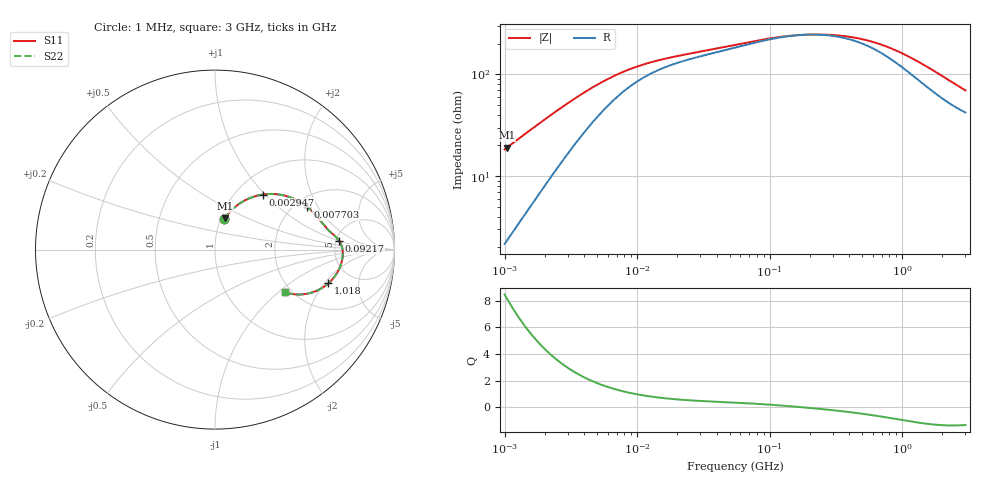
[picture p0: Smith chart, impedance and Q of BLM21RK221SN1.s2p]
! BLM21RK221SN1
# Hz S RI R 50
!Freq.(Hz) S11(Real) S11(Imag) S21(Real) S21(Imag) S12(Real) S12(Imag) S22(Real) S22(Imag)
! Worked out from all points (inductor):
!   401 points, 1 MHz to 3 GHz, reference 50 ohm
!   read as one part in series: L = 2.87 uH near 1.041 MHz
!   highest Q = 8.16 at 1.041 MHz (marker M1), where L = 2.89 uH
!   self-resonance near 183.6 MHz
!   S11 on the Smith chart (normalised r, x): 1 MHz: 1.04, +0.36; 2.947 MHz: 1.32, +0.97; 7.703 MHz: 2.32, +1.63; 92.17 MHz: 5.32, +1.01; 1.018 GHz: 3.31, -2.20; 3 GHz: 1.84, -1.11
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1000000  0.0512 0.169  0.9488 -0.169  0.9488 -0.169  0.0512 0.169
1040844  0.055 0.1747  0.945 -0.1747  0.945 -0.1747  0.055 0.1747
1751453  0.1324 0.2533  0.8676 -0.2533  0.8676 -0.2533  0.1324 0.2533
2947212  0.2674 0.307  0.7326 -0.307  0.7326 -0.307  0.2674 0.307
3823119  0.346 0.3083  0.654 -0.3083  0.654 -0.3083  0.346 0.3083
5481359  0.4448 0.2808  0.5552 -0.2808  0.5552 -0.2808  0.4448 0.2808
7703107  0.5144 0.2374  0.4856 -0.2374  0.4856 -0.2374  0.5144 0.2374
1.040059e7  0.5562 0.198  0.4438 -0.198  0.4438 -0.198  0.5562 0.198
1.461624e7  0.5881 0.16  0.4119 -0.16  0.4119 -0.16  0.5881 0.16
2.459509e7  0.6214 0.1192  0.3786 -0.1192  0.3786 -0.1192  0.6214 0.1192
5.477226e7  0.6653 0.0783  0.3347 -0.0783  0.3347 -0.0783  0.6653 0.0783
9.216659e7  0.6913 0.0493  0.3087 -0.0493  0.3087 -0.0493  0.6913 0.0493
2.094008e8  0.7115 -0.0106  0.2885 0.0106  0.2885 0.0106  0.7115 -0.0106
3.002264e8  0.7108 -0.0419  0.2892 0.0419  0.2892 0.0419  0.7108 -0.0419
4.219165e8  0.7038 -0.0759  0.2962 0.0759  0.2962 0.0759  0.7038 -0.0759
5.81181e8  0.6891 -0.1133  0.3109 0.1133  0.3109 0.1133  0.6891 -0.1133
8.005644e8  0.6625 -0.1554  0.3375 0.1554  0.3375 0.1554  0.6625 -0.1554
1.017911e9  0.6316 -0.1881  0.3684 0.1881  0.3684 0.1881  0.6316 -0.1881
1.347129e9  0.5815 -0.2222  0.4185 0.2222  0.4185 0.2222  0.5815 -0.2222
1.818868e9  0.5129 -0.2459  0.4871 0.2459  0.4871 0.2459  0.5129 -0.2459
2.312676e9  0.4524 -0.2497  0.5476 0.2497  0.5476 0.2497  0.4524 -0.2497
3e9  0.3892 -0.2378  0.6108 0.2378  0.6108 0.2378  0.3892 -0.2378
